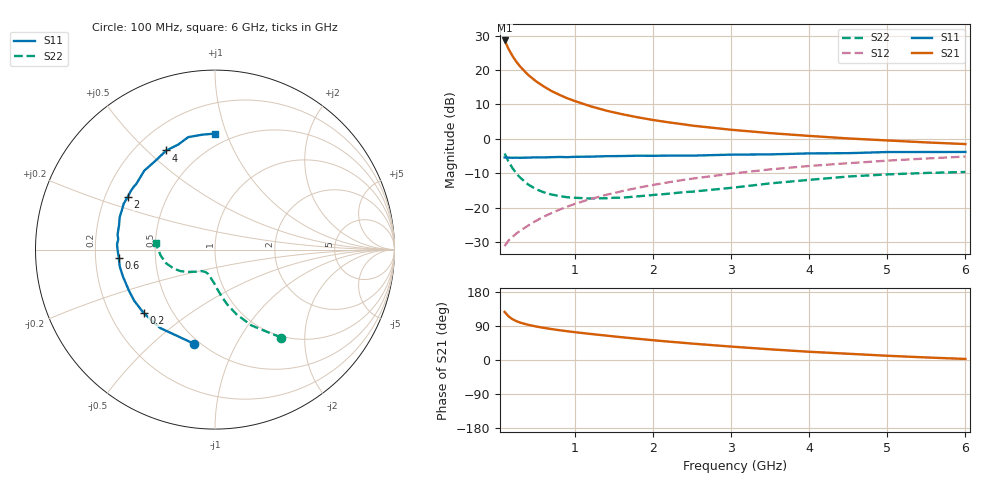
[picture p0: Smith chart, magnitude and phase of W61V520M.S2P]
! SIEMENS Small Signal Semiconductors
! BFR193W
! Si NPN RF Bipolar Junction Transistor in SOT323
! VCE = 1.5 V  IC = 20 mA
! Common Emitter S-Parameters:  September  1992
# GHz  S  MA  R  50
!  f  S11  S21  S12  S22
! GHz  MAG  ANG  MAG  ANG  MAG  ANG  MAG  ANG
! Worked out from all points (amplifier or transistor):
!   28 points, 100 MHz to 6 GHz, reference 50 ohm
!   highest |S21| = 28.6 dB at 100 MHz (marker M1)
!   |S21| within 3 dB of that: start of sweep to 163.6 MHz
!   unconditionally stable (mu >= 1): 691.2 MHz to 2.643 GHz
!   at 300 MHz: K = 0.77, MSG = 23.8 dB, |S12| = -26.7 dB
!   at 1.5 GHz: K = 1.04, MAG = 10.5 dB, |S12| = -15.7 dB
!   at 6 GHz: K = 0.92, MSG = 1.8 dB, |S12| = -5.1 dB
!   S11 on the Smith chart (normalised r, x): 100 MHz: 0.47, -0.69; 200 MHz: 0.35, -0.34; 600 MHz: 0.30, -0.04; 2 GHz: 0.30, +0.25; 4 GHz: 0.32, +0.57; 6 GHz: 0.41, +0.91
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0.1  0.5376 -102.5  26.95 126.9  0.0276 56.1  0.614 -53.0
0.15  0.5332 -125.0  20.32 115.2  0.0334 53.4  0.4682 -64.4
0.2  0.5318 -138.4  16.1 107.7  0.0376 53.3  0.3775 -71.8
0.25  0.5327 -147.5  13.23 102.6  0.0422 54.8  0.3142 -77.3
0.3  0.5313 -154.2  11.22 98.7  0.0463 56.4  0.2733 -81.0
0.4  0.5345 -163.8  8.547 92.9  0.0549 59.5  0.2181 -87.0
0.5  0.5391 -170.1  6.907 88.6  0.0642 62.1  0.1861 -91.6
0.6  0.538 -175.3  5.793 84.9  0.074 63.7  0.1677 -96.2
0.7  0.5422 -179.2  4.97 81.6  0.0835 65.1  0.1554 -99.4
0.8  0.5466 177.0  4.379 78.7  0.0934 65.9  0.1483 -102.8
0.9  0.5421 173.9  3.903 76.0  0.1034 66.3  0.1418 -105.2
1  0.5492 171.2  3.543 73.4  0.1137 66.6  0.1394 -107.6
1.2  0.5516 165.8  2.979 68.8  0.1337 66.6  0.136 -113.4
1.5  0.5618 159.5  2.425 62.2  0.1634 65.9  0.1395 -119.7
2  0.5678 149.0  1.883 52.2  0.2141 63.4  0.1529 -127.7
2.2  0.5714 145.3  1.74 48.5  0.2342 62.2  0.1596 -129.9
3  0.5905 131.9  1.358 35.4  0.3124 56.2  0.1943 -140.2
3.5  0.5952 124.2  1.213 28.2  0.3603 51.9  0.2255 -147.8
4  0.6154 116.2  1.105 21.7  0.4041 47.4  0.2539 -155.4
4.5  0.6201 109.3  1.015 16.5  0.4431 43.1  0.2839 -164.8
5.5  0.6444 96.2  0.889 6.7  0.5189 34.4  0.3201 178.4
6  0.6461 90.2  0.841 2.8  0.5536 29.7  0.3304 173.3
